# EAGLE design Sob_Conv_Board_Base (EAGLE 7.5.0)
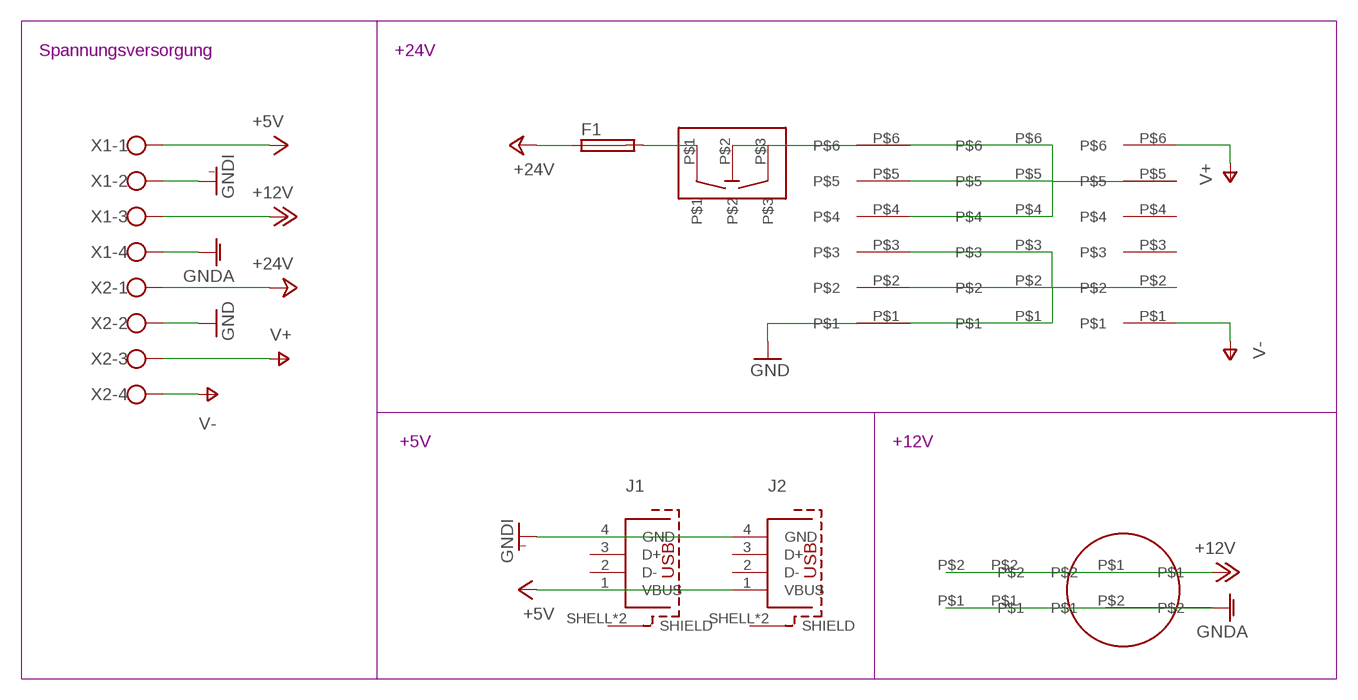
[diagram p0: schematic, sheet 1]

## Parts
F1  SH22,5A  [SH22,5A]
J1  62900416021  [62900416021]
J2  62900416021  [62900416021]
U$1  5566-2WH  [5566-2WH]
U$2  5566-2WH  [5566-2WH]
U$4  5566-6WH  [5566-6WH]
U$5  5566-6WH  [5566-6WH]
U$6  5566-6WH  [5566-6WH]
U$7  HOHLSTECKER  [HOHLSTECKER]
U$8  WIPPSCHALTER  [WIPPSCHALTER]
X1  W237-4  [W237-4]
X2  W237-4  [W237-4]

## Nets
+5V: J1.1(VBUS) J2.1(VBUS) X1.1
+12V: U$1.P$2 U$2.P$2 U$7.P$1 X1.3
+24V: F1.1 X2.1
GND: U$4.P$2 U$5.P$1 U$5.P$2 U$5.P$3 U$6.P$1 U$6.P$2 U$6.P$3 X2.2
GNDA: U$1.P$1 U$2.P$1 U$7.P$2 X1.4
GNDI: J1.4(GND) J2.4(GND) X1.2
N$2: U$4.P$5 U$5.P$4 U$5.P$5 U$5.P$6 U$6.P$4 U$6.P$5 U$6.P$6 U$8.P$2
N$3: F1.2 U$8.P$1
V+: U$4.P$6 X2.3
V-: U$4.P$1 X2.4
Unconnected: J1.2(D-) J1.3(D+) J1.SHELL1(SHIELD) J1.SHELL(SHIELD) J2.2(D-) J2.3(D+) J2.SHELL1(SHIELD) J2.SHELL(SHIELD) U$4.P$3 U$4.P$4 U$8.P$3

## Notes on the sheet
- Spannungsversorgung | +24V
- +5V | +12V

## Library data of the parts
F1 = fuse:SH22,5A: FUSE HOLDER; MPN: 0031.7701.11; OC_FARNELL: unknown; OC_NEWARK: 04F1224
J1 J2 = InputOutputIO (rev18b):62900416021: WR-COM SMT Horizontal USB Type A,4 pins=>Code : Con_I-O_COM_USB-2.0_A_62900416021 Details see: http://katalog.we-online.de/en/em/629_004_160_21 Created 2014-07-09, Karrer Zheng 2014 (C) Würth Elektronik
U$1 U$2 = 5566-2wh:5566-2WH
U$4-U$6 = 5566-6wh:5566-6WH
U$7 = hohlstecker:HOHLSTECKER
U$8 = wippschalter:WIPPSCHALTER
X1 X2 = con-wago-500:W237-4: WAGO SCREW CLAMP; OC_FARNELL: unknown; OC_NEWARK: unknown

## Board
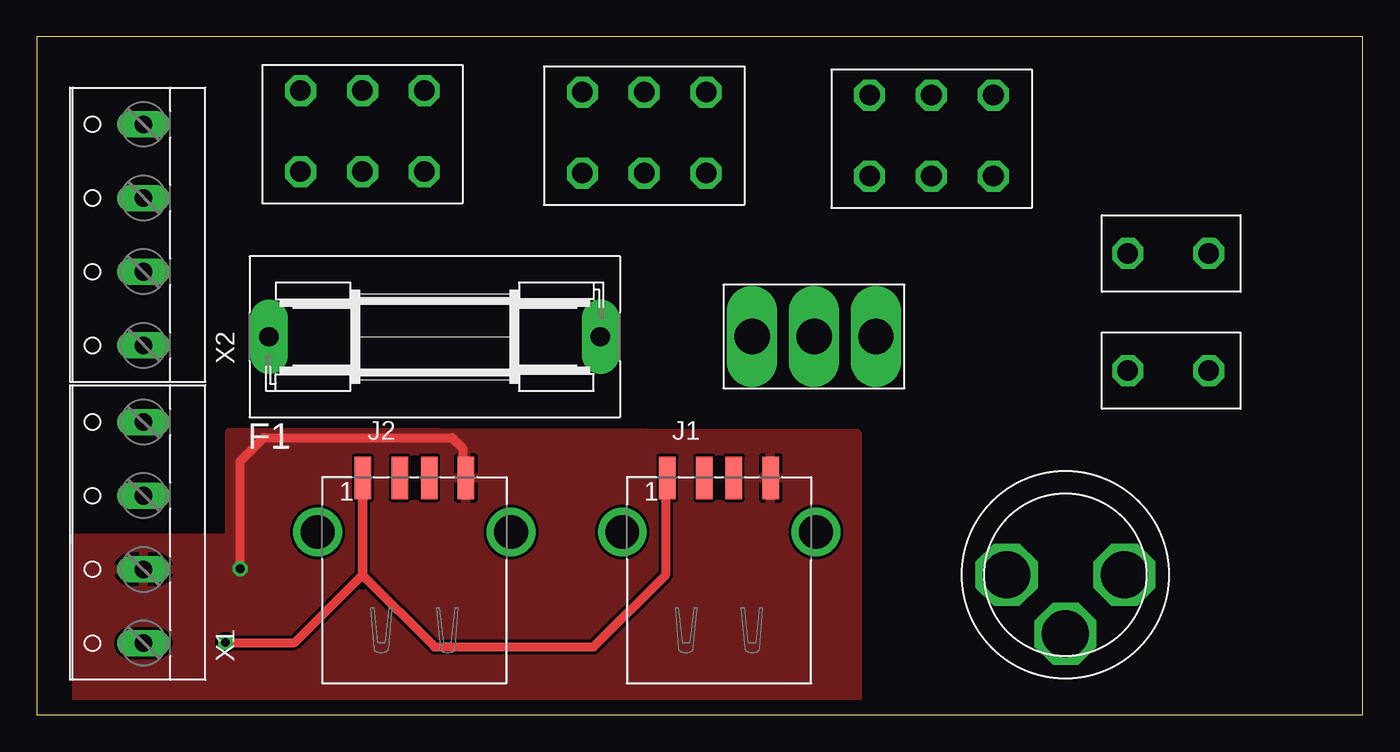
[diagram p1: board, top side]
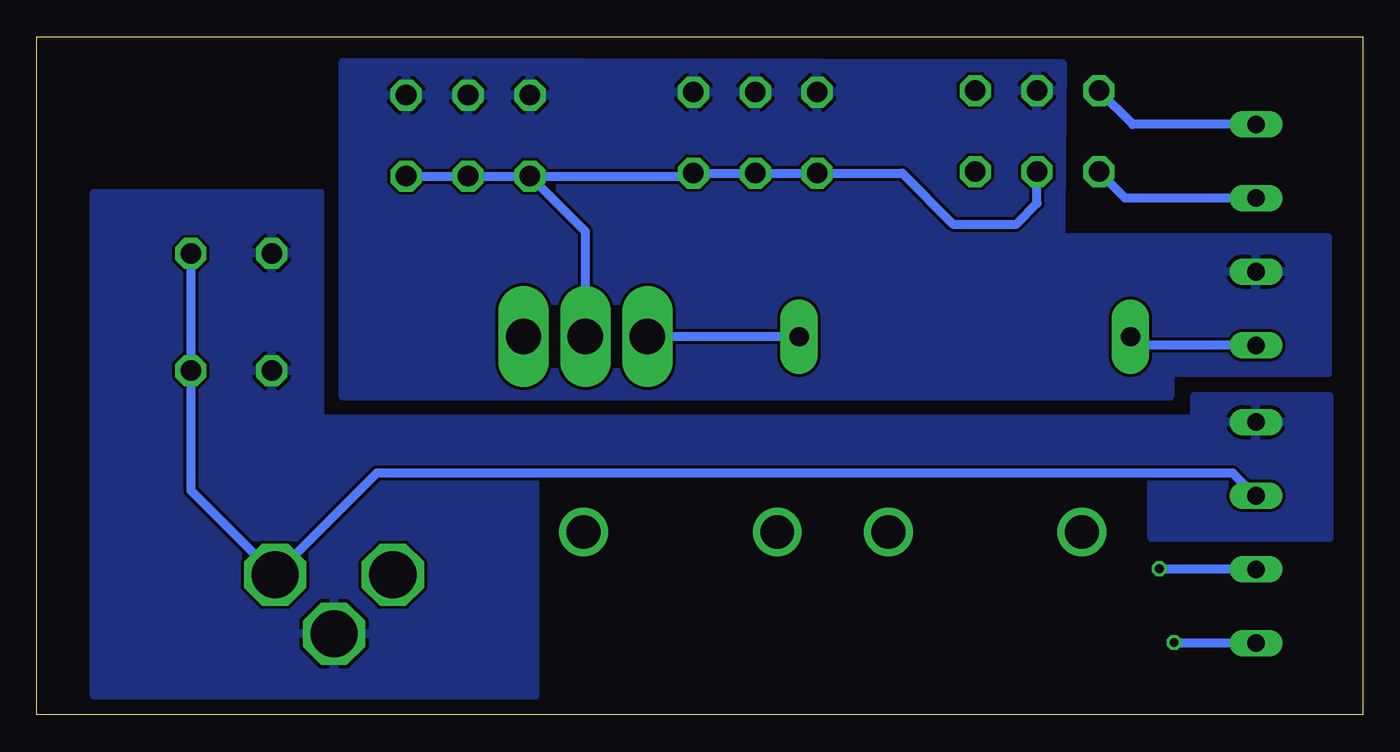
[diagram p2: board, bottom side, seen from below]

Size 90 x 46 mm. Coordinates in mm from the lower left corner, seen from the top.
Outline: 0,0 90,0 90,46 0,46 0,0
Copper layers (1*16): Top 0.035mm / dielectric 1.5mm / Bottom 0.035mm
Design rules "default": minimum track width 10mil, minimum drill 24mil, track to track 8mil, track to pad 8mil, pad to pad 8mil, via to via 8mil, smd to smd 8mil, copper to edge 40mil, drill to drill 8mil, minimum pad ring 10mil, minimum via ring 8mil, stop-mask expansion 4mil, vias tented up to drill 0mil, thermal gap 10mil

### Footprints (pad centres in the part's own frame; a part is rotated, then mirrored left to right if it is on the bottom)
SH22,5A = drill 1.321 pad 2.54 long: 1 -11.252,0; 2 11.252,0
62900416021 = smd 1.12 x 2.88: 1 -3.5,3.67; 2 -1,3.67; 3 1,3.67; 4 3.5,3.67 | drill 2.3: SHELL -6.57,0; SHELL1 6.57,0
5566-2WH = drill 1.4 octagon: P$1 0,2.75; P$2 0,-2.75
5566-6WH = drill 1.4 octagon: P$1 -4.2,2.75; P$2 0,2.75; P$3 4.2,2.75; P$4 4.2,-2.75; P$5 0,-2.75; P$6 -4.2,-2.75
HOHLSTECKER = drill 3.2 octagon: P$1 4,0; P$2 0,-4; P$3 -4,0
WIPPSCHALTER = drill 2.4 long: P$1 -4.2,0; P$2 0,0; P$3 4.2,0
W237-4 = drill 1.194 long: 1 -7.5,-1.27; 2 -2.5,-1.27; 3 2.5,-1.27; 4 7.5,-1.27

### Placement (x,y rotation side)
F1  27.01,25.65 0 top
J1  46.31,12.4 0 top
J2  25.63,12.4 0 top
U$1  76.8,31.3 90 top
U$2  76.8,23.35 90 top
U$4  22.1,39.6 0 top
U$5  41.23,39.5 0 top
U$6  60.73,39.3 0 top
U$7  69.83,9.5 0 top
U$8  52.76,25.67 0 top
X1  5.98,12.36 90 top
X2  5.98,32.56 90 top

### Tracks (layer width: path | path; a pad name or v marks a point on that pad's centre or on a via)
+5V  (via drill 0.6)
  Top 0.61: v12.8,4.9 17.5,4.9 22.1,9.5 22.1,16.04 J2.1 22.13,9.47 27,4.6 37.8,4.6 42.7,9.5 42.7,15.96 J1.1
  Bottom 0.61: X1.1 12.76,4.86 v12.8,4.9
+12V
  Bottom 0.61: X1.3 8.8,16.4 66.93,16.4 U$7.P$1 79.55,15.22 U$2.P$2 U$1.P$2
+24V
  Bottom 0.61: X2.1 15.17,25.06 F1.1
GND
  pour Bottom: 2.4,32.4 2.4,23.2 13.1,23.2 13.1,21.6 69.2,21.6 69.2,44.3 20.4,44.2 20.5,34.1 20.5,32.4
GNDA
  pour Bottom: 2.3,21.6 2.3,12 14.3,12 14.3,16 56.2,16 56.2,1.3 86.1,1.3 86.1,35.4 70.8,35.4 70.8,20.1 11.4,20.1 11.4,21.6
GNDI  (via drill 0.6)
  Top 0.61: v13.8,9.9 13.8,17.2 15.4,18.8 28.2,18.8 28.9,18.1 28.9,16.3 J2.4
  Bottom 0.61: X1.2 13.76,9.86 v13.8,9.9
  pour Top: 2.5,11.9 2.5,12 13.1,12 13.1,19.2 55.7,19.1 55.7,0.9 2.7,1 2.7,11.9
N$2
  Bottom 0.61: U$8.P$2 52.76,32.78 U$6.P$6 | U$6.P$4 U$6.P$5 U$6.P$6 | U$6.P$6 45.63,36.55 U$5.P$4 U$5.P$5 U$5.P$6 31.25,36.75 27.8,33.3 23.5,33.3 22.1,34.7 U$4.P$5
N$3
  Bottom 0.61: F1.2 48.54,25.65 U$8.P$1
V+
  Bottom 0.61: X2.3 16.11,35.06 U$4.P$6
V-
  Bottom 0.61: X2.4 15.61,40.06 U$4.P$1

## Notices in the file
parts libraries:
InputOutputIO: Copyright: Würth Elektronik
